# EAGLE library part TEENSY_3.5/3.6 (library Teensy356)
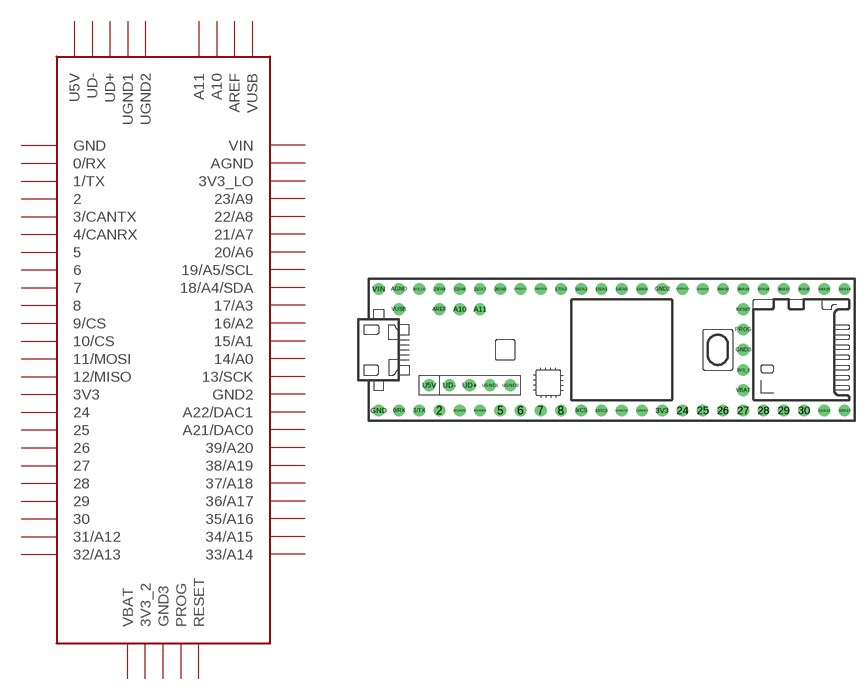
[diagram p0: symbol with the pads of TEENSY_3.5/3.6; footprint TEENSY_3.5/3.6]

Designator prefix -

## TEENSY_3.5/3.6  [TEENSY_3.5/3.6]
0/RX  0/RX
1/TX  1/TX
2  2
3/CANTX  3/CANTX
3V3  3V3
3V3_2  3V3_2
3V3_LO  3V3_LO
4/CANRX  4/CANRX
5  5
6  6
7  7
8  8
9/CS  9/CS
10/CS  10/CS
11/MOSI  11/MOSI
12/MISO  12/MISO
13/SCK  13/SCK
14/A0  14/A0
15/A1  15/A1
16/A2  16/A2
17/A3  17/A3
18/A4/SDA  18/A4/SDA
19/A5/SCL  19/A5/SCL
20/A6  20/A6
21/A7  21/A7
21/DAC0  A21/DAC0
22/A8  22/A8
23/A9  23/A9
24  24
25  25
26  26
27  27
28  28
29  29
30  30
31/A12  31/A12
32/A13  32/A13
33/A14  33/A14
34/A15  34/A15
35/A16  35/A16
36/A17  36/A17
37/A18  37/A18
38/A19  38/A19
39/A20  39/A20
A10  A10
A11  A11
A22/DAC1  A22/DAC1
AGND  AGND
AREF  AREF
GND  GND
GND2  GND2
GND3  GND3
PROG  PROG
RESET  RESET
U5V  U5V
UD+  UD+
UD-  UD-
UGND1  UGND1
UGND2  UGND2
VBAT  VBAT
VIN  VIN
VUSB  VUSB

## Footprint TEENSY_3.5/3.6 (pad centres in mm)
drill 0.965: 0/RX -25.4,-7.62; 1/TX -22.86,-7.62; 2 -20.32,-7.62; 3/CANTX -17.78,-7.62; 3V3 7.62,-7.62; 3V3_2 17.78,-2.54; 3V3_LO -22.86,7.62; 4/CANRX -15.24,-7.62; 5 -12.7,-7.62; 6 -10.16,-7.62; 7 -7.62,-7.62; 8 -5.08,-7.62; 9/CS -2.54,-7.62; 10/CS 0,-7.62; 11/MOSI 2.54,-7.62; 12/MISO 5.08,-7.62; 13/SCK 5.08,7.62; 14/A0 2.54,7.62; 15/A1 0,7.62; 16/A2 -2.54,7.62; 17/A3 -5.08,7.62; 18/A4/SDA -7.62,7.62; 19/A5/SCL -10.16,7.62; 20/A6 -12.7,7.62; 21/A7 -15.24,7.62; 21/DAC0 12.7,7.62; 22/A8 -17.78,7.62; 23/A9 -20.32,7.62; 24 10.16,-7.62; 25 12.7,-7.62; 26 15.24,-7.62; 27 17.78,-7.62; 28 20.32,-7.62; 29 22.86,-7.62; 30 25.4,-7.62; 31/A12 27.94,-7.62; 32/A13 30.48,-7.62; 33/A14 30.48,7.62; 34/A15 27.94,7.62; 35/A16 25.4,7.62; 36/A17 22.86,7.62; 37/A18 20.32,7.62; 38/A19 17.78,7.62; 39/A20 15.24,7.62; A10 -17.78,5.08; A11 -15.24,5.08; A22/DAC1 10.16,7.62; AGND -25.4,7.62; AREF -20.32,5.08; GND -27.94,-7.62; GND2 7.62,7.62; GND3 17.78,0; PROG 17.78,2.54; RESET 17.78,5.08; U5V -21.59,-4.445; UD+ -16.51,-4.445; UD- -19.05,-4.445; UGND1 -13.97,-4.445; UGND2 -11.43,-4.445; VBAT 17.78,-5.08; VIN -27.94,7.62; VUSB -25.4,5.08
